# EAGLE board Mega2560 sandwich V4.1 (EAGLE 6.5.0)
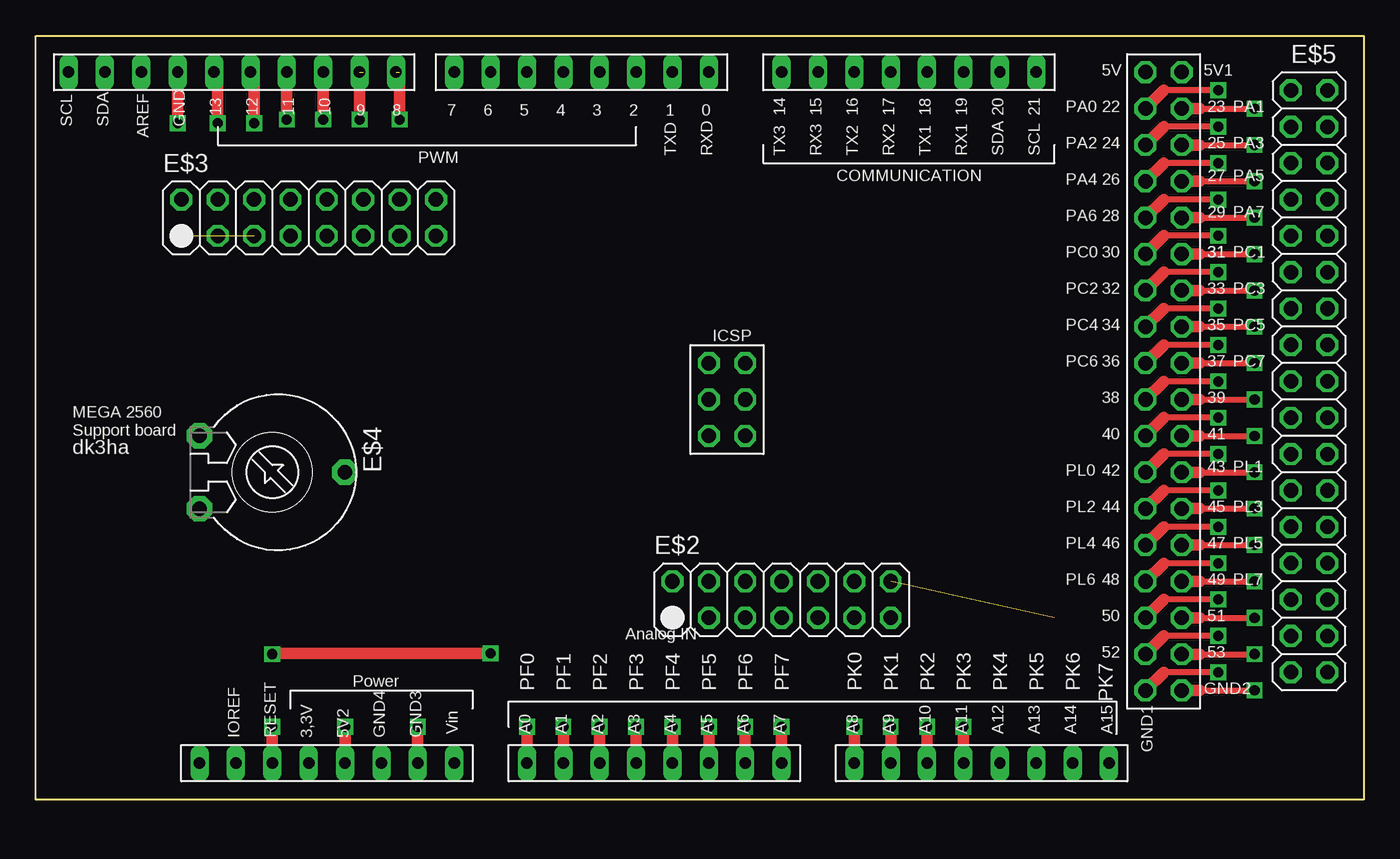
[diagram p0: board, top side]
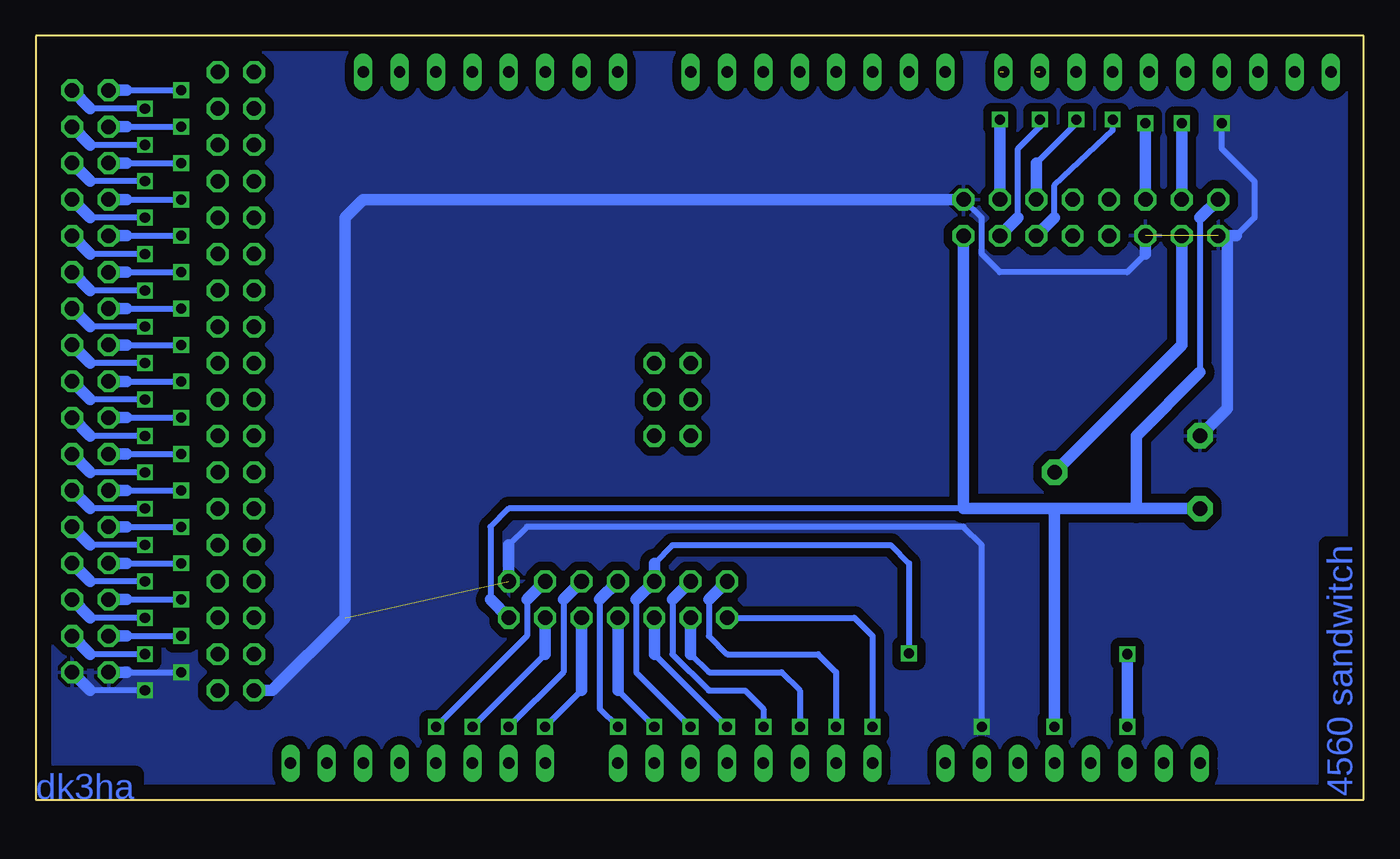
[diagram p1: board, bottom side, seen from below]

Size 92.71 x 53.34 mm. Coordinates in mm from the lower left corner, seen from the top.
Copper layers (1*16): Top 0.035mm / dielectric 1.5mm / Bottom 0.035mm
Design rules "default": minimum track width 10mil, minimum drill 24mil, track to track 8mil, track to pad 8mil, pad to pad 8mil, via to via 8mil, smd to smd 8mil, copper to edge 40mil, drill to drill 8mil, minimum pad ring 10mil, minimum via ring 8mil, stop-mask expansion 4mil, vias tented up to drill 0mil, thermal gap 10mil

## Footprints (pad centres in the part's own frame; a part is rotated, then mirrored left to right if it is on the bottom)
FOOTPRINTMEGA2560 = drill 0.8 long: 0 46.99,50.8; 1 44.45,50.8; 2 41.91,50.8; 3 39.37,50.8; 3,3V 19.05,2.54; 4 36.83,50.8; 5 34.29,50.8; 5V2 21.59,2.54; 6 31.75,50.8; 7 29.21,50.8; 8 25.146,50.8; 9 22.606,50.8; 10 20.066,50.8; 11 17.526,50.8; 12 14.986,50.8; 13 12.446,50.8; 14 52.07,50.8; 15 54.61,50.8; 16 57.15,50.8; 17 59.69,50.8; 18 62.23,50.8; 19 64.77,50.8; 20 67.31,50.8; 21 69.85,50.8; A0 34.29,2.54; A1 36.83,2.54; A2 39.37,2.54; A3 41.91,2.54; A4 44.45,2.54; A5 46.99,2.54; A6 49.53,2.54; A7 52.07,2.54; A8 57.15,2.54; A9 59.69,2.54; A10 62.23,2.54; A11 64.77,2.54; A12 67.31,2.54; A13 69.85,2.54; A14 72.39,2.54; A15 74.93,2.54; AREF 7.366,50.8; GND 9.906,50.8; GND3 26.67,2.54; GND4 24.13,2.54; IIOREF 13.97,2.54; P$1 11.43,2.54; RESET 16.51,2.54; SCL 2.286,50.8; SDA 4.826,50.8; VIN 29.21,2.54 | drill 1.016 octagon: 5V 77.47,50.8; 5V1 80.01,50.8; 22 77.47,48.26; 23 80.01,48.26; 24 77.47,45.72; 25 80.01,45.72; 26 77.47,43.18; 27 80.01,43.18; 28 77.47,40.64; 29 80.01,40.64; 30 77.47,38.1; 31 80.01,38.1; 32 77.47,35.56; 33 80.01,35.56; 34 77.47,33.02; 35 80.01,33.02; 36 77.47,30.48; 37 80.01,30.48; 38 77.47,27.94; 39 80.01,27.94; 40 77.47,25.4; 41 80.01,25.4; 42 77.47,22.86; 43 80.01,22.86; 44 77.47,20.32; 45 80.01,20.32; 46 77.47,17.78; 47 80.01,17.78; 48 77.47,15.24; 49 80.01,15.24; 50 77.47,12.7; 51 80.01,12.7; 52 77.47,10.16; 53 80.01,10.16; GND1 77.47,7.62; GND2 80.01,7.62; P$87 46.99,30.48; P$88 49.53,30.48; P$89 46.99,27.94; P$90 49.53,27.94; P$91 46.99,25.4; P$92 49.53,25.4
2X07 = drill 1.016 octagon: 1 -7.62,-1.27; 2 -7.62,1.27; 3 -5.08,-1.27; 4 -5.08,1.27; 5 -2.54,-1.27; 6 -2.54,1.27; 7 0,-1.27; 8 0,1.27; 9 2.54,-1.27; 10 2.54,1.27; 11 5.08,-1.27; 12 5.08,1.27; 13 7.62,-1.27; 14 7.62,1.27
2X08 = drill 1.016 octagon: 1 -8.89,-1.27; 2 -8.89,1.27; 3 -6.35,-1.27; 4 -6.35,1.27; 5 -3.81,-1.27; 6 -3.81,1.27; 7 -1.27,-1.27; 8 -1.27,1.27; 9 1.27,-1.27; 10 1.27,1.27; 11 3.81,-1.27; 12 3.81,1.27; 13 6.35,-1.27; 14 6.35,1.27; 15 8.89,-1.27; 16 8.89,1.27
PT-10 = drill 1.016 pad 1.778 octagon: 1 -2.54,-5.08; 2 2.54,-5.08; 3 0,5.08
2X17 = drill 1.016 octagon: 1 -20.32,-1.27; 2 -20.32,1.27; 3 -17.78,-1.27; 4 -17.78,1.27; 5 -15.24,-1.27; 6 -15.24,1.27; 7 -12.7,-1.27; 8 -12.7,1.27; 9 -10.16,-1.27; 10 -10.16,1.27; 11 -7.62,-1.27; 12 -7.62,1.27; 13 -5.08,-1.27; 14 -5.08,1.27; 15 -2.54,-1.27; 16 -2.54,1.27; 17 0,-1.27; 18 0,1.27; 19 2.54,-1.27; 20 2.54,1.27; 21 5.08,-1.27; 22 5.08,1.27; 23 7.62,-1.27; 24 7.62,1.27; 25 10.16,-1.27; 26 10.16,1.27; 27 12.7,-1.27; 28 12.7,1.27; 29 15.24,-1.27; 30 15.24,1.27; 31 17.78,-1.27; 32 17.78,1.27; 33 20.32,-1.27; 34 20.32,1.27

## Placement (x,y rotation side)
E$1  [FOOTPRINTMEGA2560]  0,0 0 top
E$2  [2X07]  52.07,13.97 0 top
E$3  [2X08]  19.05,40.64 0 top
E$4  [PT-10]  16.51,22.86 270 top
E$5  [2X17]  88.9,29.21 270 top

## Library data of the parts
E$1 = dk3ha-2020
E$2 E$3 E$5 = pinhead+
E$4 = rcl

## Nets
GND: E$2.14 E$3.1 E$3.5 E$3.16 E$4.1 E$5.33 E$5.34
S$1: E$2.1
S$2: E$2.2
S$3: E$2.3
S$4: E$2.4
S$5: E$2.5
S$6: E$2.6
S$7: E$2.7
S$8: E$2.8
S$9: E$2.9
S$10: E$2.10
S$11: E$2.11
S$12: E$2.12
S$13: E$5.1
S$14: E$2.13 E$3.2 E$3.15 E$4.2
S$15: E$5.2
S$16: E$5.3
S$17: E$3.3 E$4.3
S$18: E$3.4
S$19: E$5.4
S$20: E$3.6
S$21: E$3.11
S$22: E$3.12
S$23: E$3.13
S$24: E$3.14
S$25: E$5.5
S$26: E$5.6
S$27: E$5.7
S$28: E$5.8
S$29: E$5.9
S$30: E$5.10
S$31: E$5.11
S$32: E$5.12
S$33: E$5.13
S$34: E$5.14
S$35: E$5.15
S$36: E$5.16
S$37: E$5.17
S$38: E$5.18
S$39: E$5.19
S$40: E$5.20
S$41: E$5.21
S$42: E$5.22
S$43: E$5.23
S$44: E$5.24
S$45: E$5.25
S$46: E$5.26
S$47: E$5.27
S$48: E$5.28
S$49: E$5.29
S$50: E$5.30
S$51: E$5.31
S$52: E$5.32

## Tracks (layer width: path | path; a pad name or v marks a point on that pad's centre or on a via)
GND  (via drill 0.7)  (2 unrouted)
  Top 0.406: v82.55,8.89 78.74,8.89 | 81.28,7.62 v85.09,7.62
  Top 0.813: v9.91,47.24 9.91,50.8 | 26.67,2.54 v26.67,5.08 | 78.74,8.89 v77.47,7.62 | 80.01,7.62 81.28,7.62
  Bottom 0.406: v9.91,47.24 9.91,45.47 7.62,43.18 7.62,40.64 8.89,39.37 | 15.24,38.1 16.51,36.83 25.4,36.83 26.67,38.1 26.67,40.64 E$3.16 | v26.67,5.08 26.67,17.78 27.94,19.05 58.42,19.05 59.69,17.78 | 86.36,8.89 v82.55,8.89 | v85.09,7.62 88.9,7.62
  Bottom 0.813: E$4.1 9.53,27.3 9.53,39.37 E$3.1 8.89,39.37 | E$3.5 15.24,38.1 | E$3.16 69.85,41.91 71.12,40.64 71.12,12.7 76.2,7.62 v77.47,7.62 | E$2.14 59.69,17.78 | E$5.33 86.36,8.89 | 88.9,7.62 E$5.34
  pour Bottom (isolate 0.61): 92.71,53.34 92.71,0 0,0 0,53.34
S$1  (via drill 0.7)
  Top 0.813: v34.29,5.08 34.29,2.54
  Bottom 0.406: E$2.1 35.56,12.7 34.29,11.43 v34.29,5.08
S$2  (via drill 0.7)
  Top 0.813: v36.83,5.08 36.83,2.54
  Bottom 0.406: 45.72,13.97 45.72,11.43 44.45,10.16 38.1,10.16 36.83,8.89 v36.83,5.08
  Bottom 0.813: E$2.2 45.72,13.97
S$3  (via drill 0.7)
  Top 0.813: v39.37,5.08 39.37,2.54
  Bottom 0.406: 46.99,10.16 45.72,8.89 40.64,8.89 39.37,7.62 v39.37,5.08
  Bottom 0.813: E$2.3 46.99,10.16
S$4  (via drill 0.7)
  Top 0.813: v41.91,5.08 41.91,2.54
  Bottom 0.406: 48.26,13.97 48.26,10.16 45.72,7.62 43.18,7.62 41.91,6.35 v41.91,5.08
  Bottom 0.813: E$2.4 48.26,13.97
S$5  (via drill 0.7)
  Top 0.813: v44.45,5.08 44.45,2.54
  Bottom 0.406: 49.53,10.16 v44.45,5.08
  Bottom 0.813: E$2.5 49.53,10.16
S$6  (via drill 0.7)
  Top 0.406: 16.51,10.22 v16.51,10.16
  Top 0.813: v46.99,5.08 46.99,2.54 | v31.75,10.22 16.51,10.22 | v16.51,5.08 16.51,2.54
  Bottom 0.406: 50.8,13.97 50.8,8.89 v46.99,5.08 | 49.53,16.51 48.26,17.78 33.02,17.78 31.75,16.51 v31.75,10.22
  Bottom 0.813: 50.8,13.97 E$2.6 49.53,16.51 | v16.51,10.16 v16.51,5.08
S$7  (via drill 0.7)
  Top 0.813: v49.53,5.08 49.53,2.54
  Bottom 0.406: 52.07,7.62 v49.53,5.08
  Bottom 0.813: E$2.7 52.07,7.62
S$8  (via drill 0.7)
  Top 0.813: v52.07,5.08 52.07,2.54
  Bottom 0.406: 53.34,13.97 53.34,6.35 v52.07,5.08
  Bottom 0.813: E$2.8 53.34,13.97
S$9  (via drill 0.7)
  Top 0.813: v57.15,5.08 57.15,2.54
  Bottom 0.406: 54.61,7.62 v57.15,5.08
  Bottom 0.813: E$2.9 54.61,7.62
S$10  (via drill 0.7)
  Top 0.813: v59.69,5.08 59.69,2.54
  Bottom 0.406: 55.88,13.97 55.88,8.89 v59.69,5.08
  Bottom 0.813: E$2.10 55.88,13.97
S$11  (via drill 0.7)
  Top 0.813: v62.23,5.08 62.23,2.54
  Bottom 0.406: 57.15,10.16 v62.23,5.08
  Bottom 0.813: E$2.11 57.15,10.16
S$12  (via drill 0.7)
  Top 0.813: v64.77,5.08 64.77,2.54
  Bottom 0.406: 58.42,13.97 58.42,11.43 v64.77,5.08
  Bottom 0.813: E$2.12 58.42,13.97
S$13  (via drill 0.7)
  Top 0.406: v82.55,49.53 78.74,49.53
  Top 0.813: 78.74,49.53 77.47,48.26
  Bottom 0.406: 86.36,49.53 v82.55,49.53
  Bottom 0.813: E$5.1 86.36,49.53
S$14  (via drill 0.7)
  Top 0.813: 21.59,2.54 v21.59,5.08
  Bottom 0.406: 11.43,40.64 11.43,29.84 | 27.94,20.32 59.69,20.32 60.96,19.05 60.96,13.97
  Bottom 0.813: E$3.2 11.43,40.64 | v21.59,5.08 21.59,20.32 | 21.59,20.32 27.94,20.32 E$3.15 | 60.96,13.97 E$2.13 | E$4.2 15.88,20.32 | 15.88,20.32 21.59,20.32 | 11.43,29.84 15.88,25.4 15.88,20.32
S$15  (via drill 0.7)
  Top 0.406: 81.28,48.26 v85.09,48.26
  Top 0.813: 80.01,48.26 81.28,48.26
  Bottom 0.406: v85.09,48.26 88.9,48.26
  Bottom 0.813: 88.9,48.26 E$5.2
S$16  (via drill 0.7)
  Top 0.406: v82.55,46.99 78.74,46.99
  Top 0.813: 78.74,46.99 77.47,45.72
  Bottom 0.406: 86.36,46.99 v82.55,46.99
  Bottom 0.813: E$5.3 86.36,46.99
S$17
  Bottom 0.813: E$4.3 12.7,31.75 E$3.3
S$18  (via drill 0.7)
  Top 0.813: v12.7,47.24 12.7,50.55 12.45,50.8
  Bottom 0.813: E$3.4 v12.7,47.24
S$19  (via drill 0.7)
  Top 0.406: 81.28,45.72 v85.09,45.72
  Top 0.813: 80.01,45.72 81.28,45.72
  Bottom 0.406: v85.09,45.72 88.9,45.72
  Bottom 0.813: 88.9,45.72 E$5.4
S$20  (via drill 0.7)
  Top 0.813: 14.99,50.8 15.24,50.55 v15.24,47.24
  Bottom 0.813: v15.24,47.24 E$3.6
S$21  (via drill 0.7)
  Top 0.813: v17.53,47.5 17.53,50.8
  Bottom 0.406: 21.59,40.64 21.59,42.93 17.53,46.74 v17.53,47.5
  Bottom 0.813: E$3.11 21.59,40.64
S$22  (via drill 0.7)
  Top 0.813: v20.07,47.5 20.07,50.8
  Bottom 0.406: 22.86,44.45 20.07,47.24 v20.07,47.5
  Bottom 0.813: E$3.12 22.86,44.45
S$23  (via drill 0.7)  (1 unrouted)
  Top 0.813: v22.61,47.5 v22.61,50.8
  Bottom 0.406: 24.13,40.64 24.13,45.47 22.61,46.99 v22.61,47.5
  Bottom 0.813: E$3.13 24.13,40.64
S$24  (via drill 0.7)  (1 unrouted)
  Top 0.813: v25.4,47.5 25.4,50.55 25.15,50.8
  Bottom 0.813: E$3.14 v25.4,47.5
S$25  (via drill 0.7)
  Top 0.406: v82.55,44.45 78.74,44.45
  Top 0.813: 78.74,44.45 77.47,43.18
  Bottom 0.406: 86.36,44.45 v82.55,44.45
  Bottom 0.813: E$5.5 86.36,44.45
S$26  (via drill 0.7)
  Top 0.406: 81.28,43.18 v85.09,43.18
  Top 0.813: 80.01,43.18 81.28,43.18
  Bottom 0.406: v85.09,43.18 88.9,43.18
  Bottom 0.813: 88.9,43.18 E$5.6
S$27  (via drill 0.7)
  Top 0.406: v82.55,41.91 78.74,41.91
  Top 0.813: 78.74,41.91 77.47,40.64
  Bottom 0.406: 86.36,41.91 v82.55,41.91
  Bottom 0.813: E$5.7 86.36,41.91
S$28  (via drill 0.7)
  Top 0.406: 81.28,40.64 v85.09,40.64
  Top 0.813: 80.01,40.64 81.28,40.64
  Bottom 0.406: v85.09,40.64 88.9,40.64
  Bottom 0.813: 88.9,40.64 E$5.8
S$29  (via drill 0.7)
  Top 0.406: v82.55,39.37 78.74,39.37
  Top 0.813: 78.74,39.37 77.47,38.1
  Bottom 0.406: 86.36,39.37 v82.55,39.37
  Bottom 0.813: E$5.9 86.36,39.37
S$30  (via drill 0.7)
  Top 0.406: 81.28,38.1 v85.09,38.1
  Top 0.813: 80.01,38.1 81.28,38.1
  Bottom 0.406: v85.09,38.1 88.9,38.1
  Bottom 0.813: 88.9,38.1 E$5.10
S$31  (via drill 0.7)
  Top 0.406: v82.55,36.83 78.74,36.83
  Top 0.813: 78.74,36.83 77.47,35.56
  Bottom 0.406: 86.36,36.83 v82.55,36.83
  Bottom 0.813: E$5.11 86.36,36.83
S$32  (via drill 0.7)
  Top 0.406: 81.28,35.56 v85.09,35.56
  Top 0.813: 80.01,35.56 81.28,35.56
  Bottom 0.406: v85.09,35.56 88.9,35.56
  Bottom 0.813: 88.9,35.56 E$5.12
S$33  (via drill 0.7)
  Top 0.406: v82.55,34.29 78.74,34.29
  Top 0.813: 78.74,34.29 77.47,33.02
  Bottom 0.406: 86.36,34.29 v82.55,34.29
  Bottom 0.813: E$5.13 86.36,34.29
S$34  (via drill 0.7)
  Top 0.406: 81.28,33.02 v85.09,33.02
  Top 0.813: 80.01,33.02 81.28,33.02
  Bottom 0.406: v85.09,33.02 88.9,33.02
  Bottom 0.813: 88.9,33.02 E$5.14
S$35  (via drill 0.7)
  Top 0.406: v82.55,31.75 78.74,31.75
  Top 0.813: 78.74,31.75 77.47,30.48
  Bottom 0.406: 86.36,31.75 v82.55,31.75
  Bottom 0.813: E$5.15 86.36,31.75
S$36  (via drill 0.7)
  Top 0.406: 81.28,30.48 v85.09,30.48
  Top 0.813: 80.01,30.48 81.28,30.48
  Bottom 0.406: v85.09,30.48 88.9,30.48
  Bottom 0.813: 88.9,30.48 E$5.16
S$37  (via drill 0.7)
  Top 0.406: v82.55,29.21 78.74,29.21
  Top 0.813: 78.74,29.21 77.47,27.94
  Bottom 0.406: 86.36,29.21 v82.55,29.21
  Bottom 0.813: E$5.17 86.36,29.21
S$38  (via drill 0.7)
  Top 0.406: 81.28,27.94 v85.09,27.94
  Top 0.813: 80.01,27.94 81.28,27.94
  Bottom 0.406: v85.09,27.94 88.9,27.94
  Bottom 0.813: 88.9,27.94 E$5.18
S$39  (via drill 0.7)
  Top 0.406: v82.55,26.67 78.74,26.67
  Top 0.813: 78.74,26.67 77.47,25.4
  Bottom 0.406: 86.36,26.67 v82.55,26.67
  Bottom 0.813: E$5.19 86.36,26.67
S$40  (via drill 0.7)
  Top 0.406: 81.28,25.4 v85.09,25.4
  Top 0.813: 80.01,25.4 81.28,25.4
  Bottom 0.406: v85.09,25.4 88.9,25.4
  Bottom 0.813: 88.9,25.4 E$5.20
S$41  (via drill 0.7)
  Top 0.406: v82.55,24.13 78.74,24.13
  Top 0.813: 78.74,24.13 77.47,22.86
  Bottom 0.406: 86.36,24.13 v82.55,24.13
  Bottom 0.813: E$5.21 86.36,24.13
S$42  (via drill 0.7)
  Top 0.406: 81.28,22.86 v85.09,22.86
  Top 0.813: 80.01,22.86 81.28,22.86
  Bottom 0.406: v85.09,22.86 88.9,22.86
  Bottom 0.813: 88.9,22.86 E$5.22
S$43  (via drill 0.7)
  Top 0.406: v82.55,21.59 78.74,21.59
  Top 0.813: 78.74,21.59 77.47,20.32
  Bottom 0.406: 86.36,21.59 v82.55,21.59
  Bottom 0.813: E$5.23 86.36,21.59
S$44  (via drill 0.7)
  Top 0.406: 81.28,20.32 v85.09,20.32
  Top 0.813: 80.01,20.32 81.28,20.32
  Bottom 0.406: v85.09,20.32 88.9,20.32
  Bottom 0.813: 88.9,20.32 E$5.24
S$45  (via drill 0.7)
  Top 0.406: v82.55,19.05 78.74,19.05
  Top 0.813: 78.74,19.05 77.47,17.78
  Bottom 0.406: 86.36,19.05 v82.55,19.05
  Bottom 0.813: E$5.25 86.36,19.05
S$46  (via drill 0.7)
  Top 0.406: 81.28,17.78 v85.09,17.78
  Top 0.813: 80.01,17.78 81.28,17.78
  Bottom 0.406: v85.09,17.78 88.9,17.78
  Bottom 0.813: 88.9,17.78 E$5.26
S$47  (via drill 0.7)
  Top 0.406: v82.55,16.51 78.74,16.51
  Top 0.813: 78.74,16.51 77.47,15.24
  Bottom 0.406: 86.36,16.51 v82.55,16.51
  Bottom 0.813: E$5.27 86.36,16.51
S$48  (via drill 0.7)
  Top 0.406: 81.28,15.24 v85.09,15.24
  Top 0.813: 80.01,15.24 81.28,15.24
  Bottom 0.406: v85.09,15.24 88.9,15.24
  Bottom 0.813: 88.9,15.24 E$5.28
S$49  (via drill 0.7)
  Top 0.406: v82.55,13.97 78.74,13.97
  Top 0.813: 78.74,13.97 77.47,12.7
  Bottom 0.406: 86.36,13.97 v82.55,13.97
  Bottom 0.813: E$5.29 86.36,13.97
S$50  (via drill 0.7)
  Top 0.406: 81.28,12.7 v85.09,12.7
  Top 0.813: 80.01,12.7 81.28,12.7
  Bottom 0.406: v85.09,12.7 88.9,12.7
  Bottom 0.813: 88.9,12.7 E$5.30
S$51  (via drill 0.7)
  Top 0.406: v82.55,11.43 78.74,11.43
  Top 0.813: 78.74,11.43 77.47,10.16
  Bottom 0.406: 86.36,11.43 v82.55,11.43
  Bottom 0.813: E$5.31 86.36,11.43
S$52  (via drill 0.7)
  Top 0.406: 81.28,10.16 v85.09,10.16
  Top 0.813: 80.01,10.16 81.28,10.16
  Bottom 0.406: v85.09,10.16 88.9,10.16
  Bottom 0.813: 88.9,10.16 E$5.32

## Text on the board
Bottom: 4560 sandwitch | dk3ha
